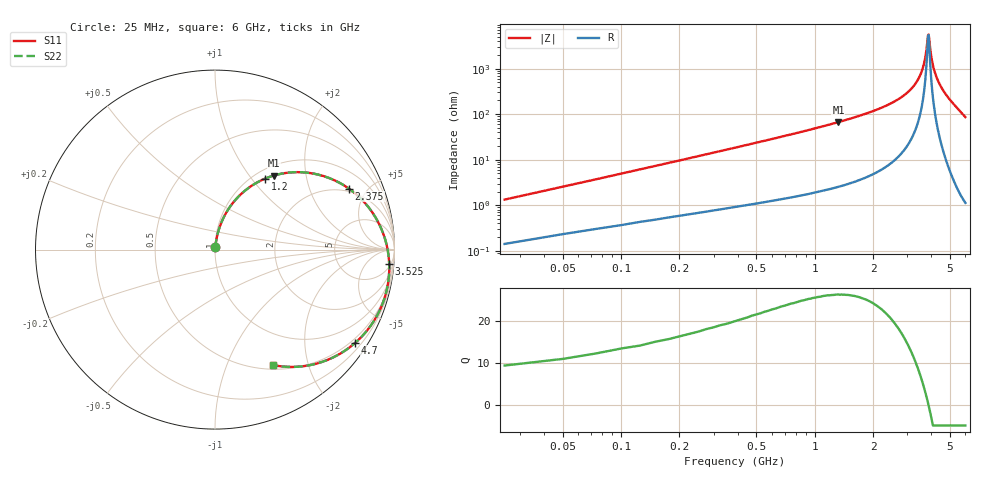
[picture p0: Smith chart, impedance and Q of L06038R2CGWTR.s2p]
!	AVX Thin Film Operation
!	Date:	March	2003
!	Description: Accu-L® Series Thin Film SMD RF Inductors
!	Part Number: L06038R2CGWTR
!	25MHz-6GHz
!	Serial	Measurements
#	mhz	S	db	R	50
!	S11	S11	S21	S21	S12	S12	S22	S22
!	dB	Phase	dB	Phase	dB	Phase	dB	Phase
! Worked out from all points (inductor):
!   240 points, 25 MHz to 6 GHz, reference 50 ohm
!   read as one part in series: L = 7.97 nH near 50 MHz
!   highest Q = 26.3 at 1.325 GHz (marker M1), where L = 8.04 nH
!   self-resonance near 3.85 GHz
!   S11 on the Smith chart (normalised r, x): 25 MHz: 1.00, +0.03; 1.2 GHz: 1.13, +1.17; 2.375 GHz: 1.83, +3.79; 3.525 GHz: 7, -22; 4.7 GHz: 0.38, -3.27; 6 GHz: 0.55, -1.48
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25  -37.95 82.7  -0.01 -0.8  -0.01 -0.8  -37.95 82.7
50  -32.33 83.0  -0.02 -1.5  -0.02 -1.5  -32.33 83.0
100  -26.65 82.5  -0.04 -3.0  -0.04 -3.0  -26.65 82.5
175  -22.03 81.0  -0.07 -5.1  -0.07 -5.1  -22.03 81.0
275  -18.28 78.7  -0.13 -7.9  -0.13 -7.9  -18.28 78.7
575  -12.19 71.2  -0.37 -16.1  -0.37 -16.1  -12.19 71.2
1025  -7.54 59.5  -1.00 -28.1  -1.00 -28.1  -7.54 59.5
1200  -6.33 54.9  -1.34 -32.7  -1.34 -32.7  -6.33 54.9
1325  -5.58 51.6  -1.61 -36.0  -1.61 -36.0  -5.58 51.6
2025  -2.65 33.4  -3.77 -54.0  -3.77 -54.0  -2.65 33.4
2375  -1.72 24.4  -5.38 -62.7  -5.38 -62.7  -1.72 24.4
3025  -0.63 7.9  -10.10 -78.0  -10.10 -78.0  -0.63 7.9
3300  -0.36 0.9  -13.48 -83.5  -13.48 -83.5  -0.36 0.9
3525  -0.23 -4.8  -17.83 -86.2  -17.83 -86.2  -0.23 -4.8
3725  -0.16 -9.8  -25.17 -80.9  -25.17 -80.9  -0.16 -9.8
3850  -0.15 -12.9  -34.96 -30.7  -34.96 -30.7  -0.15 -12.9
3875  -0.15 -13.5  -35.26 -0.7  -35.26 -0.7  -0.15 -13.5
4025  -0.16 -17.2  -24.22 57.9  -24.22 57.9  -0.16 -17.2
4275  -0.24 -23.3  -16.39 61.3  -16.39 61.3  -0.24 -23.3
4700  -0.56 -33.6  -10.45 54.2  -10.45 54.2  -0.56 -33.6
5025  -0.94 -41.3  -7.81 47.4  -7.81 47.4  -0.94 -41.3
6000  -2.85 -63.3  -3.42 26.5  -3.42 26.5  -2.85 -63.3
